[IBIS VER]   5.0
[File Name]   am13e230pdt.ibs
[File Rev]   1.0
[Date]   February 08, 2026
[Source]   File originated at Texas Instruments
[Copyright]   (c) 2012, Texas Instruments Inc.
[Component]   am13e230pdt
[Manufacturer] Texas Instruments
[Package]
| Variable   Typ   Min   Max
   R_pkg 3.45E-01 2.14E-01 4.20E-01
   L_pkg 1.05E-08 9.21E-09 1.24E-08
   C_pkg 1.31E-14 1.03E-14 3.27E-14
[Pin]   signal_name   model_name   R_pin   L_pin   C_pin
   1   PC2   BCF3385DSHYPBFZSD_87U 3.78E-01 1.20E-08 2.74E-14
   2   PC3   BCF3385DSHYPBFZSD_87U 3.62E-01 1.17E-08 1.34E-14
   3   PC4   BCF3385DSHYPBFZSD_87U 3.56E-01 1.15E-08 1.31E-14
   4   PC5   BCF3385DSHYPBFZSD_87U 3.51E-01 1.13E-08 1.29E-14
   5   PC6   BCF3385DSWHYPBFZSD_87U 3.46E-01 1.11E-08 1.26E-14
   6   VDD   NC   3.49E-01 1.09E-08 1.25E-14
   7   PB13   BCF3385DSWHYPBFZSD_87U 3.41E-01 1.07E-08 1.22E-14
   8   PB14   BCF3385DSHYPBFZSD_87U 3.39E-01 1.05E-08 1.20E-14
   9   PB15   BCF3385DSHYPBFZSD_87U 3.38E-01 1.04E-08 1.18E-14
   10   PC19   BCF3385DSHYPBFZSD_87U 3.37E-01 1.02E-08 1.15E-14
   11   PC20   BCF3385DSHYPBFZSD_87U 3.37E-01 1.00E-08 1.13E-14
   12   VSS   NC 3.42E-01 9.94E-09 1.12E-14
   13   VDD   NC 3.43E-01 9.79E-09 1.10E-14
   14   PC21   BCF3385DSHYPBFZSD_87U 3.40E-01 9.60E-09 1.07E-14
   15   PC23   BCF3385DSHYPBFZSD_87U 3.42E-01 9.47E-09 1.05E-14
   16   PC24   BCF3385DSHYPBFZSD_87U 3.45E-01 9.34E-09 1.04E-14
   17   PC25   BCF3385DSHYPBFZSD_87U 3.47E-01 9.37E-09 1.04E-14
   18   PC26   BCF3385DSHYPBFZSD_87U 3.49E-01 9.54E-09 1.06E-14
   19 PC16_X1   BCF3385DSHYPBFZSD_87U 3.61E-01 9.82E-09 1.09E-14
   20 PC17_X2   BCF3385DSHYPBFZSD_87U 3.59E-01 9.95E-09 1.11E-14
   21 PD10_NRST   BQ0491FSSD_XRSN_87U 3.50E-01 1.00E-08 1.12E-14
   22   PB0   BCF3385DSHYPBFZSD_87U 3.53E-01 1.02E-08 1.15E-14
   23   PB1   BCF3385DSWHYPBFZSD_87U 3.56E-01 1.04E-08 1.17E-14
   24   PB2   BCF3385DSHYPBFZSD_87U 3.60E-01 1.06E-08 1.19E-14
   25   PB3   BCF3385DSHYPBFZSD_87U 3.65E-01 1.08E-08 1.22E-14
   26   PC18   BCF3385DSHYPBFZSD_87U 3.50E-01 1.08E-08 1.23E-14
   27   PA0   BCF3385DSWHYPBFZSD_87U 3.54E-01 1.10E-08 1.25E-14
   28   PA1   BCF3385DSHYPBFZSD_87U 3.58E-01 1.12E-08 1.27E-14
   29   PA2   BCF3385DSWHYPBFZSD_87U 3.64E-01 1.14E-08 1.30E-14
   30   VSSA   NC 2.14E-01 1.00E-08 1.58E-14
   31   VDDA   NC 2.17E-01 1.02E-08 1.60E-14
   32   PA3   BCF3385DSHYPBFZSD_87U 3.77E-01 1.20E-08 2.74E-14
   33   PA4   BCF3385DSHYPBFZSD_87U 3.84E-01 1.21E-08 2.75E-14
   34   PA5   BCF3385DSHYPBFZSD_87U 3.75E-01 1.18E-08 1.35E-14
   35   PA6   BCF3385DSHYPBFZSD_87U 3.67E-01 1.16E-08 1.32E-14
   36   PA7   BCF3385DSHYPBFZSD_87U 3.60E-01 1.14E-08 1.30E-14
   37   PB4   BCF3385DSHYPBFZSD_87U 3.54E-01 1.11E-08 1.27E-14
   38   PB5   BCF3385DSWHYPBFZSD_87U 3.49E-01 1.09E-08 1.25E-14
   39   PA16   BCF3385DSHYPBFZSD_87U 3.45E-01 1.07E-08 1.22E-14
   40   PA17   BCF3385DSHYPBFZSD_87U 3.41E-01 1.05E-08 1.20E-14
   41   PA18   BCF3385DSHYPBFZSD_87U 3.37E-01 1.03E-08 1.17E-14
   42   VREFLO   NC 3.39E-01 1.02E-08 1.16E-14
   43   VREFHI   NC 3.41E-01 1.01E-08 1.14E-14
   44   VREFHI   NC 3.41E-01 1.01E-08 1.14E-14
   45   VDDA   NC 3.41E-01 9.77E-09 1.10E-14
   46   VSS   NC 3.42E-01 9.62E-09 1.07E-14
   47   VDD   NC 3.40E-01 9.45E-09 1.05E-14
   48   PC27   BCF3385DSHYPBFZSD_87U 3.33E-01 9.23E-09 1.03E-14
   49   PC28   BCF3385DSHYPBFZSD_87U 3.32E-01 9.21E-09 1.03E-14
   50   PC29   BCF3385DSHYPBFZSD_87U 3.30E-01 9.35E-09 1.05E-14
   51   PC30   BCF3385DSHYPBFZSD_87U 3.29E-01 9.49E-09 1.07E-14
   52   PC31   BCF3385DSHYPBFZSD_87U 3.29E-01 9.64E-09 1.09E-14
   53   PC7   BCF3385DSHYPBFZSD_87U 3.29E-01 9.80E-09 1.11E-14
   54   PC8   BCF3385DSHYPBFZSD_87U 3.30E-01 9.96E-09 1.13E-14
   55   PC9   BCF3385DSHYPBFZSD_87U 3.31E-01 1.01E-08 1.15E-14
   56   PC10   BCF3385DSHYPBFZSD_87U 3.33E-01 1.03E-08 1.17E-14
   57   PC11   BCF3385DSHYPBFZSD_87U 3.36E-01 1.05E-08 1.19E-14
   58   PC12   BCF3385DSHYPBFZSD_87U 3.40E-01 1.07E-08 1.22E-14
   59   PC13   BCF3385DSHYPBFZSD_87U 3.45E-01 1.09E-08 1.24E-14
   60   PC14   BCF3385DSHYPBFZSD_87U 3.50E-01 1.11E-08 1.27E-14
   61   PC15   BCF3385DSHYPBFZSD_87U 3.56E-01 1.13E-08 1.29E-14
   62   PA26   BCF3385DSHYPBFZSD_87U 3.63E-01 1.15E-08 1.32E-14
   63   VSS   NC 2.14E-01 1.02E-08 1.59E-14
   64   VDD   NC 3.76E-01 1.20E-08 2.74E-14
   65   PA27   BCF3385DSHYPBFZSD_87U 3.73E-01 1.20E-08 2.73E-14
   66   PA28   BCF3385DSHYPBFZSD_87U 3.67E-01 1.17E-08 1.34E-14
   67   PA29   BCF3385DSHYPBFZSD_87U 3.61E-01 1.15E-08 1.32E-14
   68   PA30   BCF3385DSHYPBFZSD_87U 3.56E-01 1.13E-08 1.29E-14
   69   PA31   BCF3385DSHYPBFZSD_87U 3.52E-01 1.11E-08 1.27E-14
   70   PB24   BCF3385DSHYPBFZSD_87U 3.50E-01 1.09E-08 1.25E-14
   71   PB25   BCF3385DSHYPBFZSD_87U 3.47E-01 1.08E-08 1.22E-14
   72   PB26   BCF3385DSHYPBFZSD_87U 3.45E-01 1.06E-08 1.20E-14
   73   PB27   BCF3385DSHYPBFZSD_87U 3.43E-01 1.04E-08 1.18E-14
   74   PB28   BCF3385DSHYPBFZSD_87U 3.42E-01 1.02E-08 1.16E-14
   75   PB29   BCF3385DSHYPBFZSD_87U 3.41E-01 1.01E-08 1.14E-14
   76   PB30   BCF3385DSHYPBFZSD_87U 3.40E-01 9.91E-09 1.11E-14
   77   PB31   BCF3385DSHYPBFZSD_87U 3.39E-01 9.75E-09 1.09E-14
   78   VSS   NC 3.45E-01 9.65E-09 1.08E-14
   79   VDD   NC 3.45E-01 9.50E-09 1.06E-14
   80   PB6   BCF3385DSHYPBFZSD_87U 3.41E-01 9.31E-09 1.03E-14
   81   PB7   BCF3385DSHYPBFZSD_87U 3.42E-01 9.32E-09 1.03E-14
   82   PD0   BCF3385DSHYPBFZSD_87U 3.43E-01 9.48E-09 1.05E-14
   83   PD1   BCF3385DSHYPBFZSD_87U 3.44E-01 9.64E-09 1.08E-14
   84   PD2   BCF3385DSHYPBFZSD_87U 3.46E-01 9.82E-09 1.10E-14
   85   PD3   BCF3385DSHYPBFZSD_87U 3.48E-01 1.00E-08 1.12E-14
   86   PD4   BCF3385DSHYPBFZSD_87U 3.52E-01 1.02E-08 1.14E-14
   87   PB8   BCF3385DSHYPBFZSD_87U 3.55E-01 1.04E-08 1.17E-14
   88   PB9   BCF3385DSHYPBFZSD_87U 3.60E-01 1.06E-08 1.19E-14
   89   PA8   BCF3385DSHYPBFZSD_87U 3.64E-01 1.08E-08 1.22E-14
   90   PA9   BCF3385DSHYPBFZSD_87U 3.70E-01 1.10E-08 1.24E-14
   91   PA10   BCF3385DSHYPBFZSD_87U 3.76E-01 1.12E-08 1.27E-14
   92   PA11   BCF3385DSHYPBFZSD_87U 3.67E-01 1.13E-08 1.28E-14
   93   PA12  BCPF335585DSHYPBFZSD_87U 3.73E-01 1.15E-08 1.30E-14
   94   VSS   NC 3.84E-01 1.18E-08 1.33E-14
   95   VDD   NC 2.24E-01 1.03E-08 1.62E-14
   96   PA13 BCF3385DSHYPBFZSD_TMS_87U 3.92E-01 1.21E-08 2.76E-14
   97   PC22   BCF3385DSHYPBFZSD_87U 3.95E-01 1.22E-08 2.77E-14
   98   PA14 BCF3385DSHYPBFZSD_TMS_87U 3.60E-01 1.17E-08 1.34E-14
   99   PA15  BCPF335585DSHYPBFZSD_87U 3.53E-01 1.14E-08 1.31E-14
   100   PB10   BCF3385DSHYPBFZSD_87U 3.47E-01 1.12E-08 1.29E-14
   101   PB11   BCF3385DSHYPBFZSD_87U 3.42E-01 1.10E-08 1.26E-14
   102   PB12   BCF3385DSHYPBFZSD_87U 3.38E-01 1.08E-08 1.24E-14
   103   PD5   BCF3385DSHYPBFZSD_87U 3.34E-01 1.06E-08 1.21E-14
   104   PD6   BCF3385DSHYPBFZSD_87U 3.31E-01 1.04E-08 1.19E-14
   105   PD7   BCF3385DSHYPBFZSD_87U 3.29E-01 1.03E-08 1.17E-14
   106   PD8   BCF3385DSHYPBFZSD_87U 3.28E-01 1.01E-08 1.15E-14
   107   PD9   BCF3385DSHYPBFZSD_87U 3.27E-01 9.94E-09 1.13E-14
   108   PB16   BCF3385DSHYPBFZSD_87U 3.27E-01 9.78E-09 1.11E-14
   109   PB17   BCF3385DSHYPBFZSD_87U 3.28E-01 9.64E-09 1.09E-14
   110   VSS   NC 3.35E-01 9.55E-09 1.07E-14
   111   VDD   NC 3.36E-01 9.41E-09 1.05E-14
   112   PB18  BCPF335585DSHYPBFZSD_87U 3.34E-01 9.23E-09 1.03E-14
   113   PB19   BCF3385DSWHYPBFZSD_87U 3.34E-01 9.23E-09 1.03E-14
   114   PB20   BCF3385DSHYPBFZSD_87U 3.35E-01 9.40E-09 1.05E-14
   115   PB21   BCF3385DSHYPBFZSD_87U 3.37E-01 9.57E-09 1.07E-14
   116   PB22   BCF3385DSHYPBFZSD_87U 3.40E-01 9.76E-09 1.09E-14
   117   PB23   BCF3385DSHYPBFZSD_87U 3.43E-01 9.94E-09 1.12E-14
   118   PA19  BCPF335585DSHYPBFZSD_87U 3.47E-01 1.01E-08 1.14E-14
   119   PA20   BCF3385DSHYPBFZSD_87U 3.51E-01 1.03E-08 1.16E-14
   120   PA21   BCF3385DSHYPBFZSD_87U 3.50E-01 1.05E-08 1.18E-14
   121   PA22   BCF3385DSHYPBFZSD_87U 3.55E-01 1.07E-08 1.21E-14
   122   PA23   BCF3385DSHYPBFZSD_87U 3.60E-01 1.09E-08 1.23E-14
   123   PA24   BCF3385DSHYPBFZSD_87U 3.63E-01 1.11E-08 1.26E-14
   124   PA25   BCF3385DSHYPBFZSD_87U 3.69E-01 1.13E-08 1.28E-14
   125   PC0   BCF3385DSHYPBFZSD_87U 3.76E-01 1.15E-08 1.31E-14
   126   PC1   BCF3385DSHYPBFZSD_87U 3.85E-01 1.18E-08 1.33E-14
   127   VSS   NC 2.24E-01 1.03E-08 1.62E-14
   128   VDD   NC 4.08E-01 1.23E-08 2.79E-14
| End of package information
|   Component BCF3385DSHYPBFZSD_87U
[Component] BCF3385DSHYPBFZSD_87U
[Manufacturer] Texas Instruments
[Package]
| variable   typ   min   max
R_pkg   0.0   0.0   0.0
L_pkg   0.0H   0.0H   0.0H
C_pkg   0.0F   0.0F   0.0F
[Pin]  signal_name   model_name   R_pin   L_pin   C_pin
PAD   PAD   BCF3385DSHYPBFZSD_87U
VDDS   VDDS   Power
VSS   VSS   Gnd
A   A   NC
GZ   GZ   NC
[Model Selector] BCF3385DSHYPBFZSD_87U
BCF3385DSHYPBFZSD_87U_PUPDOFF PI=1 PSEL=1
BCF3385DSHYPBFZSD_87U_PDON PI=0 PSEL=0
BCF3385DSHYPBFZSD_87U_PUON PI=0 PSEL=1
|   Component BCF3385DSHYPBFZSD_TMS_87U
[Component] BCF3385DSHYPBFZSD_TMS_87U
[Manufacturer] Texas Instruments
[Package]
| variable   typ   min   max
R_pkg   0.0   0.0   0.0
L_pkg   0.0H   0.0H   0.0H
C_pkg   0.0F   0.0F   0.0F
[Pin]  signal_name   model_name   R_pin   L_pin   C_pin
PAD   PAD   BCF3385DSHYPBFZSD_TMS_87U
VDDS   VDDS   Power
VSS   VSS   Gnd
A   A   NC
GZ   GZ   NC
[Model Selector] BCF3385DSHYPBFZSD_TMS_87U
BCF3385DSHYPBFZSD_TMS_87U_PUPDOFF PI=1 PSEL=1
BCF3385DSHYPBFZSD_TMS_87U_PDON PI=0 PSEL=0
BCF3385DSHYPBFZSD_TMS_87U_PUON PI=0 PSEL=1
|   Component BCF3385DSWHYPBFZSD_87U
[Component] BCF3385DSWHYPBFZSD_87U
[Manufacturer] Texas Instruments
[Package]
| variable   typ   min   max
R_pkg   0.0   0.0   0.0
L_pkg   0.0H   0.0H   0.0H
C_pkg   0.0F   0.0F   0.0F
[Pin]  signal_name   model_name   R_pin   L_pin   C_pin
PAD   PAD   BCF3385DSWHYPBFZSD_87U
VDDS   VDDS   Power
VSS   VSS   Gnd
A   A   NC
GZ   GZ   NC
[Model Selector] BCF3385DSWHYPBFZSD_87U
BCF3385DSWHYPBFZSD_87U_PUPDOFF PI=1 PSEL=1
BCF3385DSWHYPBFZSD_87U_PDON PI=0 PSEL=0
BCF3385DSWHYPBFZSD_87U_PUON PI=0 PSEL=1
|   Component BCPF335585DSHYPBFZSD_87U
[Component] BCPF335585DSHYPBFZSD_87U
[Manufacturer] Texas Instruments
[Package]
| variable   typ   min   max
R_pkg   0.0   0.0   0.0
L_pkg   0.0H   0.0H   0.0H
C_pkg   0.0F   0.0F   0.0F
[Pin]  signal_name   model_name   R_pin   L_pin   C_pin
PAD   PAD   BCPF335585DSHYPBFZSD_87U
VDDS   VDDS   Power
VSS   VSS   Gnd
A   A   NC
GZ   GZ   NC
[Model Selector] BCPF335585DSHYPBFZSD_87U
BCPF335585DSHYPBFZSD_87U_PUPDOFF_D0 DS=0
BCPF335585DSHYPBFZSD_87U_PUPDOFF_D1 DS=1
BCPF335585DSHYPBFZSD_87U_PDON PI=0 PSEL=0
BCPF335585DSHYPBFZSD_87U_PUON PI=0 PSEL=1
|   Component BQ0491FSSD_XRSN_87U
[Component] BQ0491FSSD_XRSN_87U
[Manufacturer] Texas Instruments
[Package]
| variable   typ   min   max
R_pkg   0.0   0.0   0.0
L_pkg   0.0H   0.0H   0.0H
C_pkg   0.0F   0.0F   0.0F
[Pin]  signal_name   model_name   R_pin   L_pin   C_pin
PAD   PAD   BQ0491FSSD_XRSN_87U
VDDS   VDDS   Power
VSS   VSS   Gnd
A   A   NC
[Model Selector] BQ0491FSSD_XRSN_87U
BQ0491FSSD_XRSN_87U_PUPDOFF PI=1
BQ0491FSSD_XRSN_87U_PUPDON PI=0
| Models and submodels in the file (15): BCF3385DSHYPBFZSD_87U_PUPDOFF (I/O), BCF3385DSHYPBFZSD_87U_PDON (Input), BCF3385DSHYPBFZSD_87U_PUON (Input), BCF3385DSHYPBFZSD_TMS_87U_PUPDOFF (I/O), BCF3385DSHYPBFZSD_TMS_87U_PDON (Input), BCF3385DSHYPBFZSD_TMS_87U_PUON (Input), BCF3385DSWHYPBFZSD_87U_PUPDOFF (I/O), BCF3385DSWHYPBFZSD_87U_PDON (Input), BCF3385DSWHYPBFZSD_87U_PUON (Input), BCPF335585DSHYPBFZSD_87U_PUPDOFF_D0 (I/O), BCPF335585DSHYPBFZSD_87U_PUPDOFF_D1 (I/O), BCPF335585DSHYPBFZSD_87U_PDON (Input), BCPF335585DSHYPBFZSD_87U_PUON (Input), BQ0491FSSD_XRSN_87U_PUPDOFF (Input), BQ0491FSSD_XRSN_87U_PUPDON (Input)
